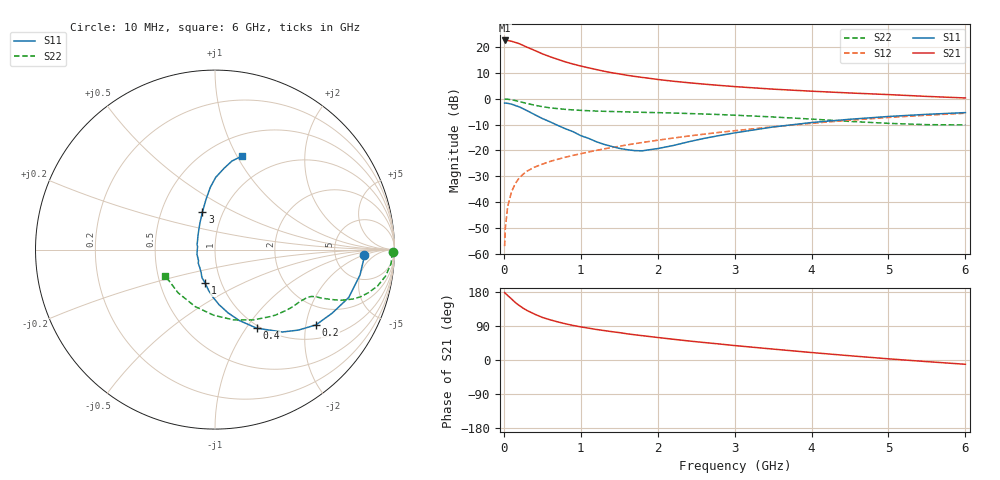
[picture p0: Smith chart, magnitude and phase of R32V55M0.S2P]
! SIEMENS Small Signal Semiconductors
! BFR181
! Si NPN RF Bipolar Junction Transistor in SOT23
! VCE = 2.5 V  IC = 5 mA
! Common Emitter S-Parameters:  May  1996
# GHz  S  MA  R  50
!  f  S11  S21  S12  S22
! GHz  MAG  ANG  MAG  ANG  MAG  ANG  MAG  ANG
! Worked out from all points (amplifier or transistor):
!   36 points, 10 MHz to 6 GHz, reference 50 ohm
!   highest |S21| = 22.6 dB at 10 MHz (marker M1)
!   |S21| within 3 dB of that: start of sweep to 332.5 MHz
!   unconditionally stable (mu >= 1): 1.103 GHz to 2.962 GHz
!   at 250 MHz: K = 0.43, MSG = 25.0 dB, |S12| = -29.2 dB
!   at 1.4 GHz: K = 1.05, MAG = 13.2 dB, |S12| = -18.9 dB
!   at 6 GHz: K = 0.86, MSG = 3.0 dB, |S12| = -5.6 dB
!   lowest NFmin = 1.55 dB at 450 MHz
!   S11 on the Smith chart (normalised r, x): 10 MHz: 10, -2; 200 MHz: 1.38, -2.28; 400 MHz: 0.97, -1.12; 1 GHz: 0.84, -0.32; 3 GHz: 0.80, +0.35; 6 GHz: 0.71, +1.05
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0.01  0.8299 -2.1  13.55 178.0  0.0014 92.2  0.9915 -0.9
0.02  0.8296 -4.0  13.46 175.9  0.0032 90.7  0.9875 -1.8
0.05  0.8203 -9.9  13.51 170.2  0.0082 85.3  0.9838 -4.6
0.1  0.7915 -19.7  13.08 161.1  0.0159 81.0  0.962 -8.8
0.15  0.7427 -28.5  12.41 151.5  0.023 74.4  0.9284 -12.6
0.2  0.7012 -36.8  11.75 143.9  0.0294 71.8  0.8891 -15.6
0.25  0.6456 -44.0  10.87 136.9  0.0346 68.4  0.852 -18.0
0.3  0.5932 -50.7  10.06 130.8  0.0397 66.9  0.8164 -19.7
0.4  0.4961 -62.0  8.7 121.0  0.0477 64.5  0.7544 -22.0
0.5  0.4168 -71.2  7.471 112.4  0.0543 63.1  0.7058 -23.2
0.6  0.3595 -78.4  6.566 106.2  0.0613 62.8  0.6718 -24.0
0.8  0.2639 -92.7  5.209 95.6  0.074 62.8  0.6269 -24.9
1  0.1938 -106.6  4.328 87.4  0.0867 63.6  0.5991 -25.8
1.1  0.1723 -115.0  4.002 84.1  0.0934 64.1  0.5896 -26.5
1.3  0.1319 -129.9  3.439 77.8  0.1073 64.3  0.5749 -27.9
1.6  0.1038 -164.6  2.87 69.2  0.1281 64.1  0.559 -30.7
2.2  0.1247 139.2  2.2 54.8  0.1739 62.7  0.5314 -37.9
3  0.2193 108.8  1.731 38.1  0.2417 58.1  0.4831 -50.6
3.5  0.2856 100.0  1.544 28.8  0.2876 54.1  0.4463 -61.4
4.5  0.4029 89.4  1.301 11.2  0.3869 43.7  0.3659 -91.1
5.5  0.5023 79.2  1.117 -4.3  0.4833 31.0  0.3166 -130.6
6  0.5422 74.0  1.042 -11.3  0.5277 23.9  0.313 -152.1
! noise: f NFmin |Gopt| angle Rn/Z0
0.45  1.55  0.48  17  0.36
0.9  1.65  0.4  35  0.34
1.8  2  0.18  88  0.34
